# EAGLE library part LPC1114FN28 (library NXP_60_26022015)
32-bit ARM Cortex-M0 microcontroller; up to 64 kB flash and 8 kB SRAM The LPC1110/11/12/13/14/15 are a ARM Cortex-M0 based, low-cost 32-bit MCU family, designed for 8/16-bit microcontroller applications, offering performance, low power, simple instruction set and memory addressing together with reduced code size compared to existing 8/16-bit architectures. The LPC1110/11/12/13/14/15 operate at CPU frequencies of up to 50 MHz. The peripheral complement of the LPC1110/11/12/13/14/15 includes up to 64 kB of flash memory, up to 8 kB of data memory, one Fast-mode Plus I 2 C-bus interface, one RS-485/EIA-485 UART, up to two SPI interfaces with SSP features, four general purpose counter/timers, a 10-bit ADC, and up to 42 general purpose I/O pins. Remark: The LPC111x series consists of the LPC1100 series (parts LPC111x/101/201/301), LPC1100L series (parts LPC111x/002/102/202/302), and the LPC1100XL series (parts LPC111x/103/203/303/323/333). The LPC1100L and LPC1100XL series include the power profiles, a windowed watchdog timer, and a configurable open-drain mode. AAL Eindhoven MK
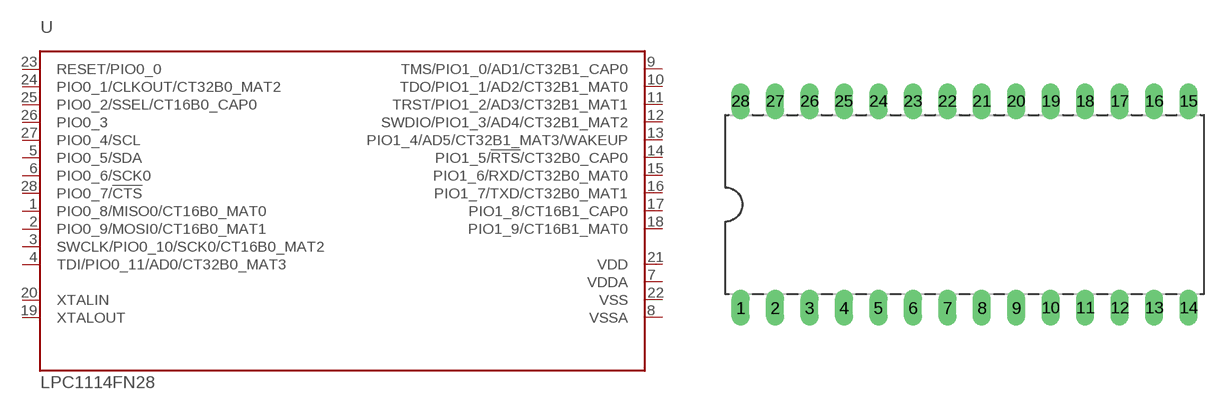
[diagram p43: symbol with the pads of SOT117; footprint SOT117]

Designator prefix U

## LPC1114FN28/102 (ADC: 6; FLASH: 32kB; GPIO: 22; PWR_PROFILES: yes; SERIES: LPC1100L; SPI: 1; SRAM: 4kB)  [SOT117]
1  PIO0_8/MISO0/CT16B0_MAT0
2  PIO0_9/MOSI0/CT16B0_MAT1
3  SWCLK/PIO0_10/SCK0/CT16B0_MAT2
4  TDI/PIO0_11/AD0/CT32B0_MAT3
5  PIO0_5/SDA
6  PIO0_6/SCK0
7  VDDA  pwr
8  VSSA  pwr
9  TMS/PIO1_0/AD1/CT32B1_CAP0
10  TDO/PIO1_1/AD2/CT32B1_MAT0
11  TRST/PIO1_2/AD3/CT32B1_MAT1
12  SWDIO/PIO1_3/AD4/CT32B1_MAT2
13  PIO1_4/AD5/CT32B1_MAT3/WAKEUP
14  PIO1_5/!RTS!/CT32B0_CAP0
15  PIO1_6/RXD/CT32B0_MAT0
16  PIO1_7/TXD/CT32B0_MAT1
17  PIO1_8/CT16B1_CAP0
18  PIO1_9/CT16B1_MAT0
19  XTALOUT  out
20  XTALIN  in
21  VDD  pwr
22  VSS  pwr
23  RESET/PIO0_0
24  PIO0_1/CLKOUT/CT32B0_MAT2
25  PIO0_2/SSEL/CT16B0_CAP0
26  PIO0_3
27  PIO0_4/SCL
28  PIO0_7/!CTS!

## Footprint SOT117 (pad centres in mm)
SOT117 DIP28: plastic dual in-line package; 28 leads (600 mil) JEDEC: MO-015 IEC: 051G05 JEITA: SC-510-28
drill 0.813 long: 1 -16.51,-7.62; 2 -13.97,-7.62; 3 -11.43,-7.62; 4 -8.89,-7.62; 5 -6.35,-7.62; 6 -3.81,-7.62; 7 -1.27,-7.62; 8 1.27,-7.62; 9 3.81,-7.62; 10 6.35,-7.62; 11 8.89,-7.62; 12 11.43,-7.62; 13 13.97,-7.62; 14 16.51,-7.62; 15 16.51,7.62; 16 13.97,7.62; 17 11.43,7.62; 18 8.89,7.62; 19 6.35,7.62; 20 3.81,7.62; 21 1.27,7.62; 22 -1.27,7.62; 23 -3.81,7.62; 24 -6.35,7.62; 25 -8.89,7.62; 26 -11.43,7.62; 27 -13.97,7.62; 28 -16.51,7.62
